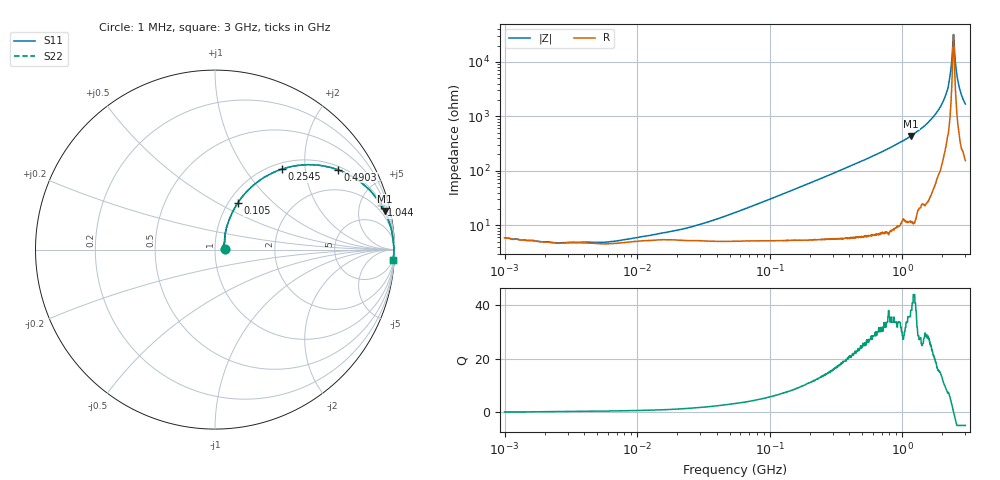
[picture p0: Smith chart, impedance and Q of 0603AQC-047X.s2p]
!s-Parameter Generated by FASTRON Sdn. Bhd.
!FASTRON P/N : 0603AQC-047X
!Keysight Technologies: E4991B_MY54100416_A.01.15
!Date: Thu Jun 25 13:54:25 2026
!Version  :Rev00  Thu Jun 25 13:54:25 2026
!Data & Calibration Information:
!Freq  S11  S21  S12  S22
!PortZ  Port1:50+j0  Port2:50+j0
!When reading reference impedance value at option line is always used.
! Remarks : This data is being provided solely for informational purposes.
# Hz S dB R 50
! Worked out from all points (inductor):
!   1601 points, 1 MHz to 3 GHz, reference 50 ohm
!   read as one part in series: L = 47.4 nH near 51.07 MHz
!   highest Q = 38.2 at 1.171 GHz (marker M1), where L = 59.5 nH
!   self-resonance near 2.431 GHz
!   S11 on the Smith chart (normalised r, x): 1 MHz: 1.12, +0.01; 105 MHz: 1.10, +0.62; 254.5 MHz: 1.11, +1.51; 490.3 MHz: 1.12, +2.98; 1.044 GHz: 1.25, +7.39; 3 GHz: 4, -33
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1000000  -25.10 3.0  -0.49 -0.2  -0.49 -0.2  -25.10 3.0
3804036  -26.60 13.5  -0.41 -0.7  -0.41 -0.7  -26.60 13.5
6729604  -26.20 23.3  -0.40 -1.2  -0.40 -1.2  -26.20 23.3
1.447069e7  -23.60 37.1  -0.47 -2.4  -0.47 -2.4  -23.60 37.1
5.504702e7  -15.80 63.9  -0.54 -8.9  -0.54 -8.9  -15.80 63.9
1.049728e8  -10.80 64.0  -0.81 -16.5  -0.81 -16.5  -10.80 64.0
2.083556e8  -5.91 54.7  -1.73 -30.3  -1.73 -30.3  -5.91 54.7
2.545267e8  -4.69 50.3  -2.26 -35.6  -2.26 -35.6  -4.69 50.3
4.902556e8  -1.77 33.1  -5.25 -54.6  -5.25 -54.6  -1.77 33.1
7.925923e8  -0.69 21.0  -8.93 -67.5  -8.93 -67.5  -0.69 21.0
1.0437e9  -0.38 15.0  -11.70 -73.1  -11.70 -73.1  -0.38 15.0
1.171007e9  -0.27 12.7  -13.10 -75.8  -13.10 -75.8  -0.27 12.7
1.596974e9  -0.10 7.0  -18.20 -80.9  -18.20 -80.9  -0.10 7.0
1.990301e9  -0.05 3.4  -24.50 -82.3  -24.50 -82.3  -0.05 3.4
2.210833e9  -0.04 1.7  -30.30 -80.2  -30.30 -80.2  -0.04 1.7
2.289646e9  -0.03 1.1  -34.50 -79.3  -34.50 -79.3  -0.03 1.1
2.371269e9  -0.03 0.5  -41.00 -69.6  -41.00 -69.6  -0.03 0.5
2.431346e9  -0.03 0.1  -49.80 -18.9  -49.80 -18.9  -0.03 0.1
2.505452e9  -0.03 -0.4  -41.60 66.8  -41.60 66.8  -0.03 -0.4
2.607784e9  -0.03 -1.1  -34.20 78.9  -34.20 78.9  -0.03 -1.1
2.700748e9  -0.04 -1.7  -30.60 80.9  -30.60 80.9  -0.04 -1.7
3e9  -0.06 -3.4  -24.60 81.4  -24.60 81.4  -0.06 -3.4
